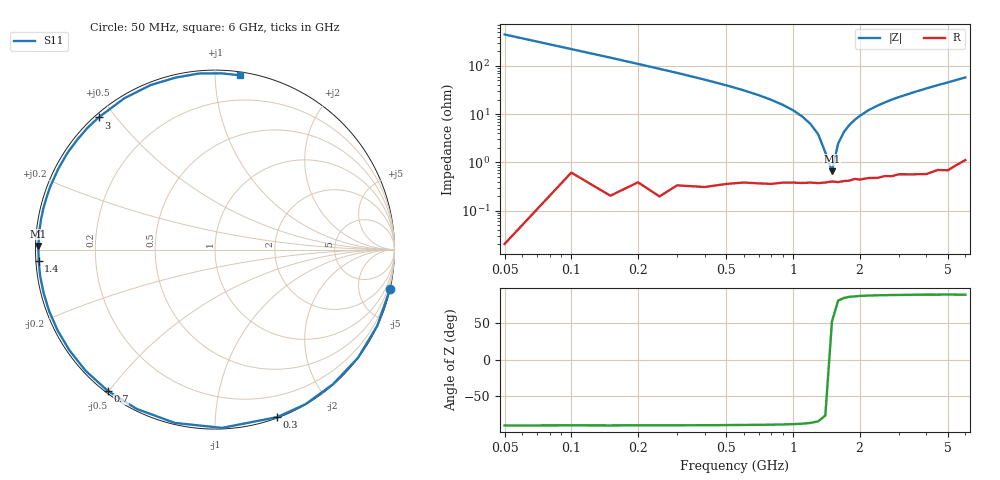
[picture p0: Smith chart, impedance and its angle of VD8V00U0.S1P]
! Infineon Technologies  Discrete & RF Semiconductors
! BBY 55-03
! Si Tuning Diode in SOD323
! VR = 8 V
! S-Parameters:  June  1999
# GHz  S  MA  R  50
!  f  S11
! GHz  MAG  ANG
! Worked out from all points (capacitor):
!   34 points, 50 MHz to 6 GHz, reference 50 ohm
!   read as one part to ground: C = 7.08 pF near 50 MHz
!   lowest |Z| = 661 mohm at 1.5 GHz (marker M1)
!   series resonance near 1.475 GHz, so ESL is about 1.6 nH
!   S11 on the Smith chart (normalised r, x): 50 MHz: 0.00, -8.99; 300 MHz: 0.01, -1.44; 700 MHz: 0.01, -0.50; 1.4 GHz: 0.01, -0.03; 3 GHz: 0.01, +0.45; 6 GHz: 0.02, +1.15
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0.05  1 -12.7
0.1  0.9988 -25.2
0.15  0.9992 -37.2
0.2  0.9974 -48.8
0.25  0.998 -59.7
0.3  0.9956 -69.7
0.4  0.9941 -87.8
0.5  0.9913 -103.1
0.6  0.989 -116.1
0.7  0.9883 -127.2
0.8  0.9877 -136.9
0.9  0.9862 -145.3
1  0.9857 -152.8
1.1  0.9856 -159.6
1.2  0.9851 -165.7
1.4  0.9848 -176.4
1.5  0.984 178.8
1.6  0.9845 174.4
1.8  0.9836 166.3
2  0.9831 159.2
2.4  0.9826 146.7
3  0.9813 131.4
3.5  0.983 120.9
4  0.9845 111.3
4.5  0.9831 102.8
5  0.9851 95.2
5.5  0.9828 88.0
6  0.981 81.8
